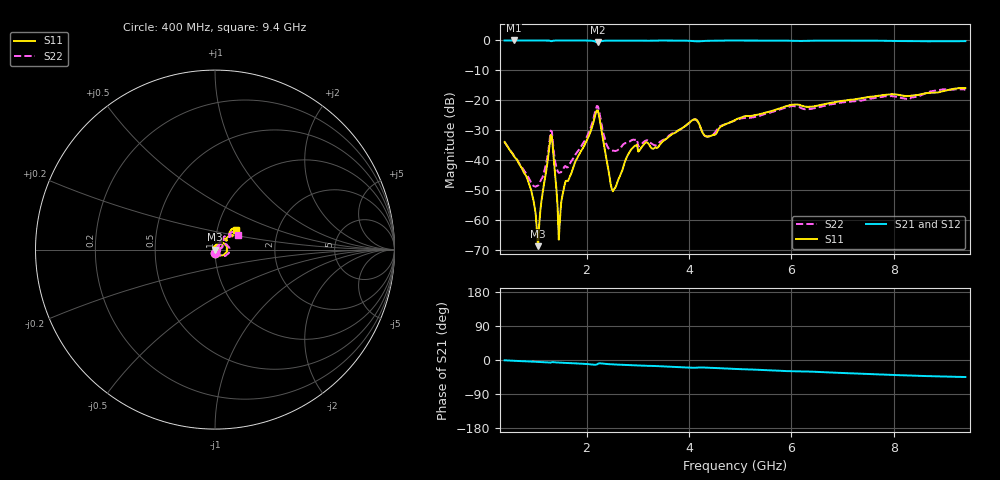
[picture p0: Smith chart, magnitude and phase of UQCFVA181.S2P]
!  Part Number  UQCFVA181  Mounting Orientation: Horizontal
!  Description: Ultra Low ESR Microwave capacitors
!  Application: Coupling, Bypass, Tuning, DC Block
!  Filters, Matching
# GHZ S DB R 50
! Freq  |S11|  S11 Ph  |S21|  S21 Ph  |S12|  S12 Ph  |S22|  S22 Ph
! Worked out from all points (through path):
!   401 points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, 400 MHz to 9.4 GHz, reference 50 ohm
!   highest |S21| = 0.00 dB at 580 MHz (marker M1); lowest = -0.7 dB at 2.223 GHz (marker M2)
!   group delay of S21, straight-line fit = 13.7 ps
!   lowest |S11| = -68.6 dB at 1.053 GHz (marker M3), VSWR 1.00, Z = 50 + j0.0103 ohm
!   |S11| at or under -10 dB: start of sweep to end of sweep
!   |S22| runs from -48.7 to -16.3 dB; largest |S21 - S12| = 0.0027
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0.4  -33.87 -87.1  -0.01 -0.8  -0.01 -0.8  -33.85 -86.5
0.58  -38.55 -88.2  0.00 -2.1  -0.01 -2.1  -38.33 -82.9
0.873  -47.67 -89.1  -0.01 -3.9  -0.01 -3.9  -45.93 -58.3
1.053  -68.60 163.9  0.00 -5.0  -0.01 -5.0  -48.39 -1.8
1.165  -48.33 92.6  -0.01 -5.7  0.00 -5.7  -44.33 34.9
1.3  -31.56 29.1  -0.21 -6.9  -0.21 -6.9  -30.07 16.2
1.345  -36.57 -53.6  -0.10 -5.7  -0.09 -5.7  -34.43 -45.9
1.435  -55.52 -90.2  -0.02 -6.7  -0.01 -6.7  -43.56 -23.4
1.48  -59.96 129.3  -0.01 -7.0  -0.01 -7.0  -44.05 -2.5
1.57  -48.29 95.8  -0.02 -7.6  -0.02 -7.6  -42.04 16.7
1.908  -36.48 90.7  -0.02 -9.7  -0.02 -9.7  -34.98 48.6
2.223  -23.49 -11.7  -0.65 -10.1  -0.65 -10.1  -21.97 -14.2
2.38  -38.73 -94.6  -0.07 -10.4  -0.07 -10.4  -34.21 -43.8
2.515  -50.29 -171.7  -0.05 -11.6  -0.05 -11.6  -36.72 -10.6
2.92  -35.56 115.0  -0.04 -13.9  -0.04 -13.9  -33.10 18.0
3.415  -35.20 67.8  -0.03 -16.3  -0.04 -16.3  -34.10 42.9
4.09  -26.38 43.3  -0.21 -20.5  -0.21 -20.5  -26.46 36.2
4.383  -32.02 41.2  -0.10 -20.4  -0.10 -20.4  -32.02 40.1
4.9  -26.54 57.9  -0.03 -23.6  -0.03 -23.5  -26.66 57.3
6.408  -22.05 41.9  -0.09 -30.8  -0.09 -30.8  -22.76 52.8
7.915  -18.00 40.6  -0.14 -39.3  -0.15 -39.4  -18.61 44.1
9.4  -15.89 43.0  -0.22 -44.9  -0.23 -45.0  -16.38 32.1
